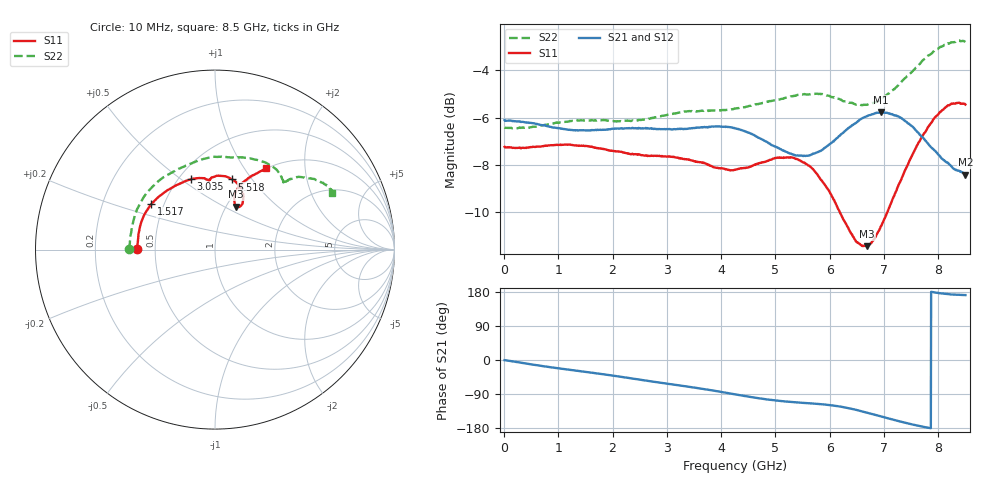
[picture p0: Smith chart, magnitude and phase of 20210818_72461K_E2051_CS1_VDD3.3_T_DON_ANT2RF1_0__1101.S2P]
!Agilent Technologies,E5071C,MY46417908,A.11.23
!Date: Wed Aug 18 14:24:19 2021
!Data & Calibration Information:
!Freq	S11:SOLT2(ON)	S21:SOLT2(ON)	S12:SOLT2(ON)	S22:SOLT2(ON)
!PortZ  Port1:50+j0  Port2:50+j0
!Above PortZ is port z conversion or system Z0 setting when saving the data.
!When reading, reference impedance value at option line is always used.
# Hz S dB R 50
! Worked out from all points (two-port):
!   1601 points, 10 MHz to 8.5 GHz, reference 50 ohm
!   highest |S21| = -5.78 dB at 6.94 GHz (marker M1); lowest = -8.4 dB at 8.5 GHz (marker M2)
!   |S21| within 3 dB of the highest: start of sweep to end of sweep
!   lowest |S11| = -11.4 dB at 6.691 GHz (marker M3), VSWR 1.73, Z = 55.6 + j28.8 ohm
!   |S11| at or under -10 dB: 6.184 GHz to 7.063 GHz (879.7 MHz wide, 13.3 % of centre)
!   |S22| runs from -6.5 to -2.7 dB; largest |S21 - S12| = 0.0022
!   S11 on the Smith chart (normalised r, x): 10 MHz: 0.39, +0.00; 1.517 GHz: 0.43, +0.27; 3.035 GHz: 0.58, +0.55; 5.518 GHz: 0.86, +0.81; 8.5 GHz: 0.99, +1.26
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1e7  -7.24 179.7  -6.11 -0.4  -6.11 -0.3  -6.41 179.6
7.847125e8  -7.19 162.9  -6.36 -17.7  -6.35 -17.7  -6.30 157.9
1.426769e9  -7.19 147.1  -6.54 -30.0  -6.54 -29.9  -6.11 138.5
1.516975e9  -7.21 144.7  -6.54 -31.7  -6.55 -31.7  -6.12 135.6
2.1325e9  -7.44 129.2  -6.46 -44.0  -6.47 -44.0  -6.15 117.8
2.843538e9  -7.63 113.0  -6.49 -59.2  -6.48 -59.2  -5.96 101.4
3.034562e9  -7.65 108.8  -6.49 -63.2  -6.48 -63.2  -5.87 97.4
3.634169e9  -7.90 98.8  -6.42 -75.7  -6.41 -75.7  -5.72 87.0
4.255e9  -8.22 94.7  -6.45 -90.6  -6.45 -90.7  -5.62 78.9
4.801544e9  -7.88 91.6  -6.99 -103.1  -6.99 -103.1  -5.37 71.6
5.236656e9  -7.69 83.4  -7.49 -110.2  -7.50 -110.1  -5.14 63.8
5.517888e9  -7.91 76.3  -7.63 -113.2  -7.64 -113.1  -5.02 58.7
5.671769e9  -8.14 72.1  -7.56 -114.6  -7.58 -114.7  -5.01 55.7
6.08035e9  -9.49 61.9  -6.97 -120.4  -6.99 -120.6  -5.13 48.7
6.467706e9  -11.19 60.1  -6.25 -130.9  -6.25 -131.0  -5.44 44.8
6.690569e9  -11.45 63.7  -5.94 -139.1  -5.93 -139.1  -5.46 43.8
6.939962e9  -10.62 68.5  -5.78 -148.7  -5.78 -148.7  -5.22 43.7
7.088538e9  -9.86 70.0  -5.82 -154.4  -5.83 -154.4  -4.98 43.5
7.422831e9  -8.07 68.3  -6.20 -166.6  -6.20 -166.7  -4.25 41.3
7.826106e9  -6.35 61.6  -7.15 -179.0  -7.12 -179.1  -3.36 35.4
8.155094e9  -5.53 58.1  -7.89 174.3  -7.86 174.3  -2.88 30.0
8.5e9  -5.45 58.2  -8.42 171.3  -8.38 171.4  -2.80 26.0
